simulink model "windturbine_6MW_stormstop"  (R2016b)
settings: Solver=VariableStepAuto  StartTime=0  StopTime=180  RelTol=1e-3
undefined symbols (not defined in the file or in its folder): c1, c2, c3, c4, c5, c6, cp_nom, Generation, lambda_nom, P_wind_base, Pelec_base, Pnom, re_lib, speed_nom, Turbine, Wind, wind_base
libraries: simulink x2

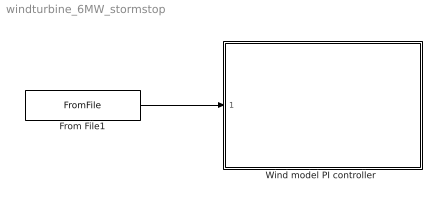
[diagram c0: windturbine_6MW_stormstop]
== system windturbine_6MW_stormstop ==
  From File1 : FromFile  Commented=on  FileName=windserie_storm3.mat  SampleTime=0
  "Wind model PI controller " : Subsystem
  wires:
  From File1/1 -> "Wind model PI controller "/1("windspeed ")

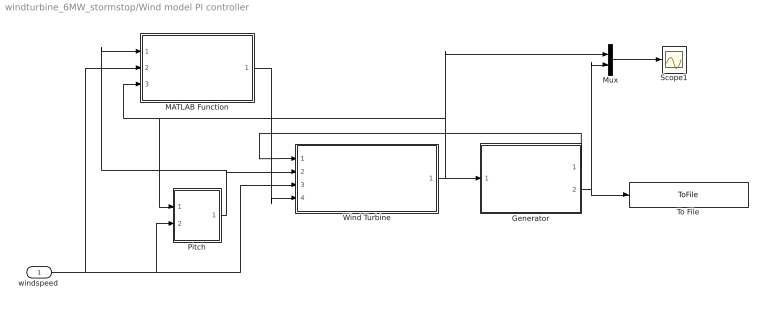
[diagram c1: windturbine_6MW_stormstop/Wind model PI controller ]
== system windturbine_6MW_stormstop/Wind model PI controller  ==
  "windspeed " : Inport
  Generator : Subsystem
  MATLAB Function : MATLAB Function  TreatAsAtomicUnit=on
  Mux : Mux  Inputs=2
  Pitch : Subsystem
  Scope1 : Scope
  To File : ToFile  Commented=on  Filename=Pwt_storm_6MW.mat  MatrixName=Pwt_storm_6MW  SaveFormat=Timeseries
  Wind Turbine : Subsystem  AncestorBlock=re_lib/Wind Generation/Wind Turbine  DialogController=POWERSYS.PowerSysDialog
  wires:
  Generator/1(w) -> Wind Turbine/1(Generator speed (pu))
  Wind Turbine/1(Tm (pu)) -> MATLAB Function/3(Tm), Pitch/1(Tm), Mux/1, Generator/1(Tm)
  Pitch/1(ß) -> Wind Turbine/2(Pitch angle (deg)), MATLAB Function/1(beta)
  Mux/1 -> Scope1/1
  Generator/2(Pe_ref) -> To File/1, Mux/2
  "windspeed "/1 -> MATLAB Function/2(windspeed), Wind Turbine/3(Wind speed (m/s)), Pitch/2(windspeed)
  MATLAB Function/1(y) -> Wind Turbine/4(Grid connect)

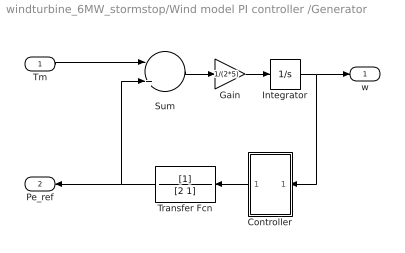
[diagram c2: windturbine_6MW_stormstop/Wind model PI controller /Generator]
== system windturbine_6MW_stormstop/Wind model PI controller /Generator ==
  Tm : Inport
  Controller : Subsystem
  Gain : Gain  Gain=1/(2*5)
  Integrator : Integrator  InitialCondition=1  LimitOutput=on  UpperSaturationLimit=2  LowerSaturationLimit=0
  Sum : Sum  Inputs=|+|-
  Transfer Fcn : TransferFcn  Denominator=[2 1]
  w : Outport
  Pe_ref : Outport  Port=2
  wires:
  Tm/1 -> Sum/1
  Sum/1 -> Gain/1
  Gain/1 -> Integrator/1
  Integrator/1 -> Controller/1(In1), w/1
  Transfer Fcn/1 -> Pe_ref/1, Sum/2
  Controller/1(Out1) -> Transfer Fcn/1

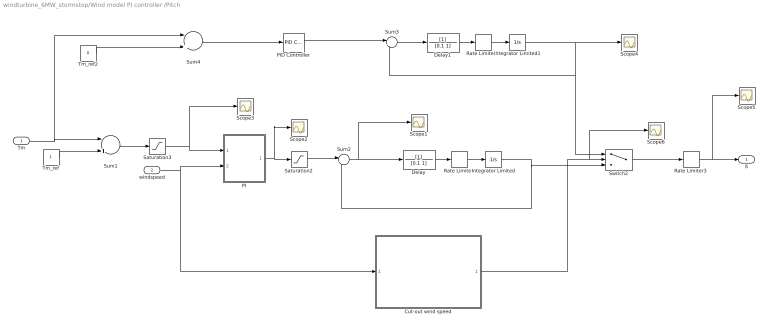
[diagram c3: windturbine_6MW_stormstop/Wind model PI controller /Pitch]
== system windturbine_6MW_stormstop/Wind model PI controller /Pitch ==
  Tm : Inport
  windspeed : Inport  Port=2
  Cut-out wind speed : MATLAB Function  TreatAsAtomicUnit=on
  Delay : TransferFcn  Denominator=[0.1 1]
  Delay1 : TransferFcn  Denominator=[0.1 1]
  Integrator Limited : Integrator  LimitOutput=on  UpperSaturationLimit=90  LowerSaturationLimit=0
  Integrator Limited1 : Integrator  LimitOutput=on  UpperSaturationLimit=60  LowerSaturationLimit=0
  PI : Subsystem
  PID Controller : simulink/Continuous/PID Controller  Controller=PI  TimeDomain=Continuous-time  SampleTime=-1  IntegratorMethod=Forward Euler  FilterMethod=Forward Euler  Form=Parallel  UseFilter=on  ControllerParametersSource=internal  P=15  I=30  D=0  N=100  InitialConditionSource=internal  InitialConditionForIntegrator=0  InitialConditionForFilter=0  ExternalReset=none  LimitOutput=on  UpperSaturationLimit=90  LowerSaturationLimit=0  LinearizeAsGain=on  AntiWindupMode=clamping  Kb=1  TrackingMode=off  Kt=1  PParamMin=[]  PParamMax=[]  IParamMin=[]  IParamMax=[]  DParamMin=[]  DParamMax=[]  NParamMin=[]  NParamMax=[]  KbParamMin=[]  KbParamMax=[]  KtParamMin=[]  KtParamMax=[]  POutMin=[]  POutMax=[]  IOutMin=[]  IOutMax=[]  DOutMin=[]  DOutMax=[]  NOutMin=[]  NOutMax=[]  KbOutMin=[]  KbOutMax=[]  KtOutMin=[]  KtOutMax=[]  IntegratorOutMin=[]  IntegratorOutMax=[]  FilterOutMin=[]  FilterOutMax=[]  SumOutMin=[]  SumOutMax=[]  SumI1OutMin=[]  SumI1OutMax=[]  SumI2OutMin=[]  SumI2OutMax=[]  SumI3OutMin=[]  SumI3OutMax=[]  SumDOutMin=[]  SumDOutMax=[]  SaturationOutMin=[]  SaturationOutMax=[]  IntegratorContinuousStateAttributes=''  IntegratorStateMustResolveToSignalObject=off  IntegratorRTWStateStorageClass=Auto  FilterContinuousStateAttributes=''  FilterStateMustResolveToSignalObject=off  FilterRTWStateStorageClass=Auto  DifferentiatorICPrevScaledInput=0  DifferentiatorOutMin=[]  DifferentiatorOutMax=[]
  Rate Limiter : RateLimiter  RisingSlewLimit=5  FallingSlewLimit=-5
  Rate Limiter1 : RateLimiter  RisingSlewLimit=5  FallingSlewLimit=-5
  Rate Limiter3 : RateLimiter  Commented=through  RisingSlewLimit=3  FallingSlewLimit=-3
  Saturation2 : Saturate  UpperLimit=90  LowerLimit=0  ZeroCross=off
  Saturation3 : Saturate  UpperLimit=1  LowerLimit=-1  ZeroCross=off
  Scope{1..6} (6 alike) : Scope
  Sum1 : Sum  Inputs=|+|-
  Sum2 : Sum  Inputs=|+-
  Sum3 : Sum  Inputs=|+-
  Sum4 : Sum  Inputs=|+|-
  Switch2 : Switch  Criteria=u2 > Threshold  ZeroCross=off
  Tm_ref : Constant
  Tm_ref2 : Constant  Value=0
  ß : Outport
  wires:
  Tm_ref/1 -> Sum1/2
  Delay/1 -> Rate Limiter/1
  Rate Limiter/1 -> Integrator Limited/1
  windspeed/1 -> Cut-out wind speed/1(windspeed), PI/2("windspeed ")
  Saturation3/1 -> PI/1(delta_w), Scope3/1
  PI/1(Out1) -> Scope2/1, Saturation2/1
  Sum2/1 -> Scope1/1, Delay/1
  Saturation2/1 -> Sum2/1
  Sum1/1 -> Saturation3/1
  Delay1/1 -> Rate Limiter1/1
  Rate Limiter1/1 -> Integrator Limited1/1
  PID Controller/1 -> Sum3/1
  Sum3/1 -> Delay1/1
  Integrator Limited1/1 -> Switch2/1, Sum3/2, Scope4/1
  Tm/1 -> Sum4/1, Sum1/1
  Tm_ref2/1 -> Sum4/2
  Sum4/1 -> PID Controller/1
  Integrator Limited/1 -> Switch2/3, Sum2/2
  Rate Limiter3/1 -> Scope5/1, ß/1
  Switch2/1 -> Rate Limiter3/1
  Cut-out wind speed/1(y) -> Scope6/1, Switch2/2

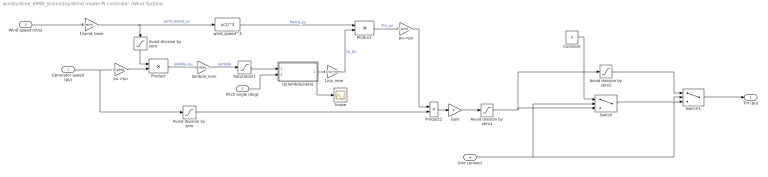
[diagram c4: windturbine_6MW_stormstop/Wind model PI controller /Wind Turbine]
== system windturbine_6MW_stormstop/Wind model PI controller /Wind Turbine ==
  Generator speed (pu) : Inport
  Pitch angle (deg) : Inport  Port=2
  Wind speed (m/s) : Inport  Port=3
  Grid connect : Inport  Port=4
  1/cp_nom : Gain  Gain=1/cp_nom
  1/wind_base : Gain  Gain=1/wind_base
  Avoid division by zero : Saturate  UpperLimit=1e6  LowerLimit=1e-6
  "Avoid division by zero " : Saturate  UpperLimit=1e6  LowerLimit=1e-6
  Avoid division by zero1 : Saturate  UpperLimit=3  LowerLimit=0
  Avoid division by zero2 : Saturate  UpperLimit=0.1  LowerLimit=-0.1
  Constant : Constant  Value=0
  Gain : Gain
  Product : Product  Inputs=/*
  "Product " : Product
  Product2 : Product  Inputs=*/
  Saturation1 : Saturate  UpperLimit=inf  LowerLimit=1e-6
  Scope : Scope
  Switch : Switch  Criteria=u2 > Threshold
  Switch1 : Switch  Criteria=u2 > Threshold  Threshold=1
  cp(lambda,beta) : Subsystem
  lambda_nom : Gain  Gain=lambda_nom
  pu->pu : Gain  Gain=P_wind_base*Pnom/Pelec_base
  "pu->pu " : Gain  Gain=1/speed_nom
  wind_speed^3 : Fcn  Expr=u(1)^3
  Tm (pu) : Outport
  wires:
  Pitch angle (deg)/1 -> cp(lambda,beta)/2(beta)
  pu->pu/1 -> Product2/1
  cp(lambda,beta)/1(cp) -> Scope/1, 1/cp_nom/1
  wind_speed^3/1 -> "Product "/1  "Pwind_pu"
  Product2/1 -> Gain/1
  Avoid division by zero/1 -> Product2/2
  Wind speed (m/s)/1 -> 1/wind_base/1
  Generator speed (pu)/1 -> Avoid division by zero/1, "pu->pu "/1
  "Product "/1 -> pu->pu/1  "Pm_pu"
  lambda_nom/1 -> Saturation1/1  "lambda"
  1/cp_nom/1 -> "Product "/2  "cp_pu"
  Saturation1/1 -> cp(lambda,beta)/1(lambda)
  Product/1 -> lambda_nom/1  "lambda_pu"
  1/wind_base/1 -> wind_speed^3/1, "Avoid division by zero "/1  "wind_speed_pu"
  "Avoid division by zero "/1 -> Product/1
  "pu->pu "/1 -> Product/2
  Avoid division by zero1/1 -> Avoid division by zero2/1, Switch/3
  Avoid division by zero2/1 -> Switch1/1
  Grid connect/1 -> Switch1/2, Switch/2
  Switch/1 -> Switch1/3
  Constant/1 -> Switch/1
  Switch1/1 -> Tm (pu)/1
  Gain/1 -> Avoid division by zero1/1

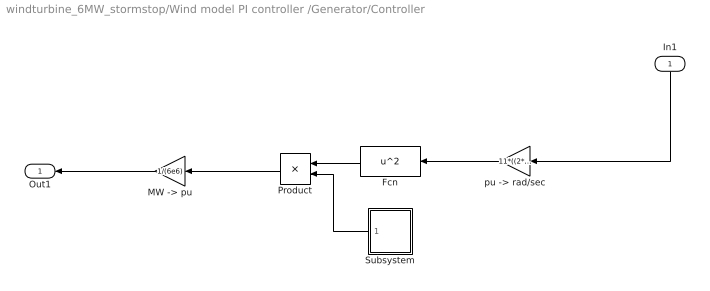
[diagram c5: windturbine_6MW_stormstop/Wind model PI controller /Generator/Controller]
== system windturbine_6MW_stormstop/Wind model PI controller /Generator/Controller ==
  In1 : Inport
  Fcn : Fcn  Expr=u^2
  "MW -> pu" : Gain  Gain=1/(6e6)
  Product : Product
  Subsystem : Subsystem
  "pu -> rad/sec" : Gain  Gain=11*((2*3.14)/60)
  Out1 : Outport
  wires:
  Product/1 -> "MW -> pu"/1
  Fcn/1 -> Product/1
  Subsystem/1(K-opt) -> Product/2
  "pu -> rad/sec"/1 -> Fcn/1
  In1/1 -> "pu -> rad/sec"/1
  "MW -> pu"/1 -> Out1/1

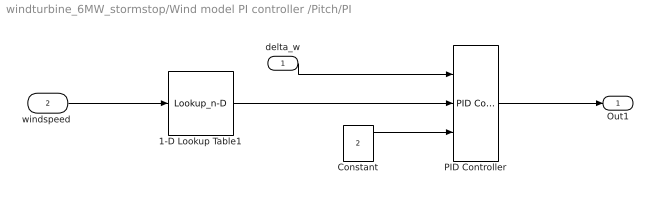
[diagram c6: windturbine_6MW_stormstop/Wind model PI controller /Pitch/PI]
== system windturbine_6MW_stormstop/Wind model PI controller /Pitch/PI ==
  delta_w : Inport
  "windspeed " : Inport  Port=2
  1-D Lookup Table1 : Lookup_n-D  NumberOfTableDimensions=1  BreakpointsForDimension1=[10,12,14,15,16,17,18,19,20,21,22,23,24,25]  Table=[20,20,20,20,20,20,20,20,15,15,15,15,15,15]  InternalRulePriority=Speed  RndMeth=Simplest
  Constant : Constant  Value=2
  PID Controller : simulink/Continuous/PID Controller  Controller=PI  TimeDomain=Continuous-time  SampleTime=-1  IntegratorMethod=Forward Euler  FilterMethod=Forward Euler  Form=Parallel  UseFilter=on  ControllerParametersSource=external  P=1  I=1  D=0  N=100  InitialConditionSource=internal  InitialConditionForIntegrator=0  InitialConditionForFilter=0  ExternalReset=none  LimitOutput=on  UpperSaturationLimit=90  LowerSaturationLimit=0  LinearizeAsGain=on  AntiWindupMode=clamping  Kb=1  TrackingMode=off  Kt=1  PParamMin=[]  PParamMax=[]  IParamMin=[]  IParamMax=[]  DParamMin=[]  DParamMax=[]  NParamMin=[]  NParamMax=[]  KbParamMin=[]  KbParamMax=[]  KtParamMin=[]  KtParamMax=[]  POutMin=[]  POutMax=[]  IOutMin=[0]  IOutMax=[]  DOutMin=[]  DOutMax=[]  NOutMin=[]  NOutMax=[]  KbOutMin=[]  KbOutMax=[]  KtOutMin=[]  KtOutMax=[]  IntegratorOutMin=[]  IntegratorOutMax=[]  FilterOutMin=[]  FilterOutMax=[]  SumOutMin=[]  SumOutMax=[]  SumI1OutMin=[]  SumI1OutMax=[]  SumI2OutMin=[]  SumI2OutMax=[]  SumI3OutMin=[]  SumI3OutMax=[]  SumDOutMin=[]  SumDOutMax=[]  SaturationOutMin=[]  SaturationOutMax=[]  IntegratorContinuousStateAttributes=''  IntegratorStateMustResolveToSignalObject=off  IntegratorRTWStateStorageClass=Auto  FilterContinuousStateAttributes=''  FilterStateMustResolveToSignalObject=off  FilterRTWStateStorageClass=Auto  DifferentiatorICPrevScaledInput=0  DifferentiatorOutMin=[]  DifferentiatorOutMax=[]
  Out1 : Outport
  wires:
  1-D Lookup Table1/1 -> PID Controller/2
  "windspeed "/1 -> 1-D Lookup Table1/1
  delta_w/1 -> PID Controller/1
  PID Controller/1 -> Out1/1
  Constant/1 -> PID Controller/3

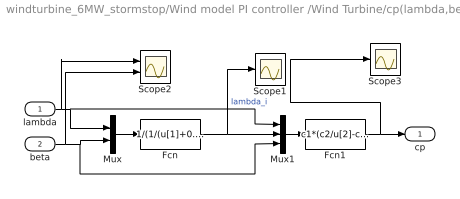
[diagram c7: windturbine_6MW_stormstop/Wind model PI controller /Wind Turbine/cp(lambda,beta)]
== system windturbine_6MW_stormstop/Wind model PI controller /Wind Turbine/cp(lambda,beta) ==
  lambda : Inport
  beta : Inport  Port=2
  Fcn : Fcn  Expr=1/(1/(u[1]+0.08*u[2])-0.035/(u[2]^3+1))
  Fcn1 : Fcn  Expr=c1*(c2/u[2]-c3*u[3]-c4)*exp(-c5/u[2])+c6*u[1]
  Mux : Mux  Inputs=2
  Mux1 : Mux  Inputs=3
  Scope1 : Scope
  Scope2 : Scope  NumInputPorts=2
  Scope3 : Scope
  cp : Outport
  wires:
  Fcn/1 -> Scope1/1, Mux1/2  "lambda_i"
  Fcn1/1 -> Scope3/1, cp/1
  lambda/1 -> Scope2/1, Mux1/1, Mux/1
  Mux1/1 -> Fcn1/1
  beta/1 -> Scope2/2, Mux1/3, Mux/2
  Mux/1 -> Fcn/1

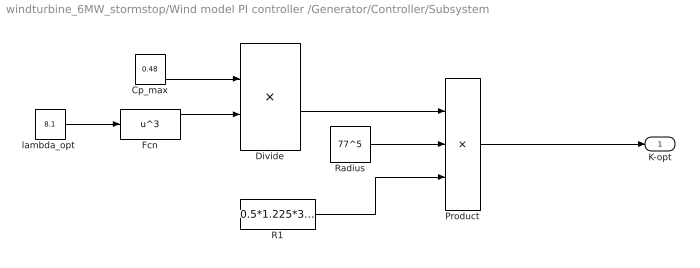
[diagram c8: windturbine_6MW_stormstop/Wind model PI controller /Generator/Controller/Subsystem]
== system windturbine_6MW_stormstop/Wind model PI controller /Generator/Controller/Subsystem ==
  Cp_max : Constant  Value=0.48
  Divide : Product  Inputs=*/
  Fcn : Fcn  Expr=u^3
  Product : Product  Inputs=3
  R1 : Constant  Value=0.5*1.225*3.14
  Radius : Constant  Value=77^5
  "lambda_opt " : Constant  Value=8.1
  K-opt : Outport
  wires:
  Divide/1 -> Product/1
  Radius/1 -> Product/2
  R1/1 -> Product/3
  Fcn/1 -> Divide/2
  "lambda_opt "/1 -> Fcn/1
  Cp_max/1 -> Divide/1
  Product/1 -> K-opt/1

== matlab function windturbine_6MW_stormstop/Wind model PI controller
/MATLAB Function ==
function y = fcn(beta, windspeed, Tm)

if (beta > 50) & (windspeed > 25) & (Tm < 0.1) 
    
    y = 1;
    
elseif (beta > 50) & (windspeed < 20) & (Tm < 0.1)
    
    y = 2;

else
    
    y = 0;
    
end

== matlab function windturbine_6MW_stormstop/Wind model PI controller
/Pitch/Cut-out wind speed ==
function y = fcn(windspeed)


if windspeed > 25

    y = 1;


% elseif windspeed > 20 & windspeed < 26 & beta > 50
%     
%     y = 1;
    
else
    
    y = 0;
    
end
